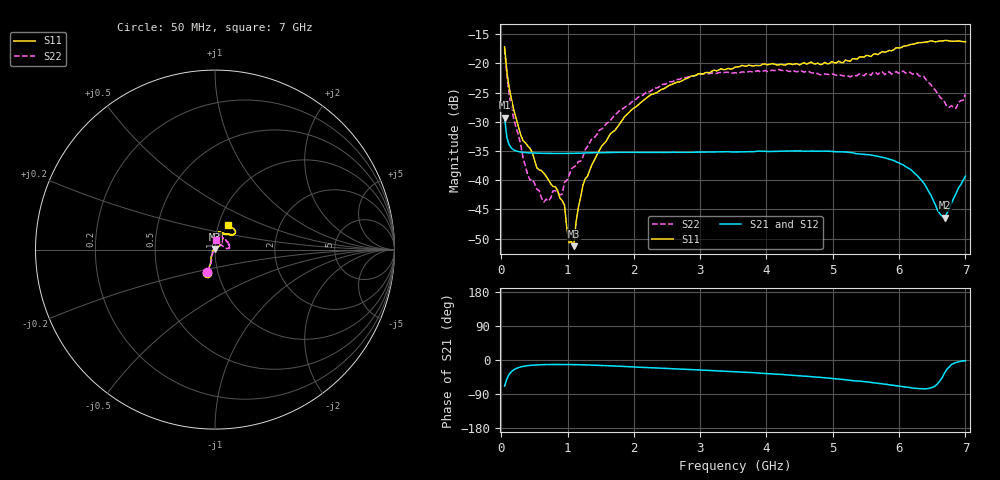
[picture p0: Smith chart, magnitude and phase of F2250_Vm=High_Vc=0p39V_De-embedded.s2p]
! Integrated Device Technology
! Corporate Headquarters
! 6024 Silver Creek Valley Road
! San Jose, CA 95138  USA
! Phone:  1-408-284-8200
! Toll Free:  1-800-223-1366
! Webpage:  http://www.idt.com/
! Timing and RF Division
! 515 Groton Road, Suite 102
! Westford, MA 01886-6024
! Device:  F2250
! Description: Voltage Variable RF Attenuator
! Frequency:  50.0 -  6000.00 MHz
! Package:  3x3 mm Thin QFN Plastic Package: 16 pin
! Ports:  2 RF, 3 DC
!  Pin  1  = GND
!  Pin  2  = NC
!  Pin  3  = RF1  = Port 1
!  Pin  4  = NC
!  Pin  5  = GND
!  Pin  6  = GND
!  Pin  7  = GND
!  Pin  8  = GND
!  Pin  9  = NC
!  Pin 10  = RF2  = Port 2
!  Pin 11  = NC
!  Pin 12  = GND
!  Pin 13  = GND
!  Pin 14  = VCNTRL
!  Pin 15  = VDD
!  Pin 16  = VMODE
! Vcntrl:  0.390 Volts
! Vmode:  +3.300 Volts
! Vdd:  +3.30  Volts
! Current:  1.261 mA
! Data:  The device was measured on a the F2250 evaluation board which has
!  individual transmission lines to the RF pins.  Data was collected
!  using a calibrated network analyzer.  The evaluation board was
!  de-embedded using a TRL calibration technique.
!  The reference plane is the edge of the package pin.
! Misc:  SN 10
!  Action Tracker AT0258
! Date Measured:  2014-11-26
! Date:  2015-10-15  MJV
! Note:
!  Integrated Device Technology supplies this data as a sample of measured
!  data at the package pin for this product.  Your particular data for this
!  product may vary.
!  Data was taken at 25 degrees C.
!  Integrated Device Technology reserves the right to change this data at anytime.
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# GHz S dB R 50
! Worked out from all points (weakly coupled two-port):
!   201 points, 50 MHz to 7 GHz, reference 50 ohm
!   highest |S21| = -29.32 dB at 50 MHz (marker M1); lowest = -46.4 dB at 6.687 GHz (marker M2)
!   lowest |S11| = -51.3 dB at 1.093 GHz (marker M3), VSWR 1.01, Z = 50 + j0.273 ohm
!   |S11| at or under -10 dB: start of sweep to end of sweep
!   |S22| runs from -43.7 to -17.6 dB; largest |S21 - S12| = 5.6e-05
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0.05  -17.18 -108.5  -29.32 -68.8  -29.32 -68.8  -17.60 -109.4
0.08475  -21.47 -107.4  -32.74 -49.5  -32.74 -49.5  -22.20 -106.3
0.189  -27.99 -120.0  -34.82 -25.8  -34.82 -25.8  -29.56 -117.9
0.328  -33.23 -134.0  -35.23 -16.9  -35.23 -16.9  -36.14 -129.9
0.43225  -34.55 -145.3  -35.33 -14.2  -35.33 -14.2  -39.97 -159.3
0.71025  -39.91 -167.6  -35.42 -12.0  -35.42 -12.0  -43.58 140.3
0.77975  -41.07 176.2  -35.42 -11.9  -35.42 -11.8  -41.84 125.0
0.91875  -43.46 156.2  -35.43 -11.9  -35.43 -11.9  -42.41 104.2
0.9535  -44.29 170.9  -35.43 -11.9  -35.43 -11.9  -40.38 104.2
1.023  -50.71 140.7  -35.42 -12.0  -35.42 -12.0  -39.20 85.6
1.0925  -51.28 88.9  -35.40 -12.1  -35.40 -12.1  -37.77 78.4
1.12725  -47.20 61.2  -35.39 -12.2  -35.39 -12.3  -37.47 70.9
1.2315  -40.86 40.5  -35.35 -12.6  -35.36 -12.6  -36.01 58.8
1.6485  -32.03 41.1  -35.27 -15.4  -35.27 -15.4  -29.78 51.2
2.37825  -24.75 46.6  -35.23 -21.4  -35.24 -21.4  -24.07 49.4
3.525  -20.66 71.7  -35.16 -31.1  -35.17 -31.1  -21.62 70.6
4.7065  -20.06 72.0  -35.02 -44.5  -35.02 -44.4  -21.66 69.0
5.85325  -17.79 40.5  -36.42 -65.3  -36.43 -65.4  -21.46 21.1
6.3745  -16.40 40.9  -40.52 -76.1  -40.53 -76.2  -22.27 4.9
6.68725  -16.11 47.8  -46.43 -34.0  -46.40 -33.9  -26.66 26.6
6.861  -16.22 54.5  -42.24 -6.3  -42.19 -6.3  -27.70 58.0
7  -16.33 62.4  -39.32 -2.1  -39.28 -2.3  -25.28 85.6
